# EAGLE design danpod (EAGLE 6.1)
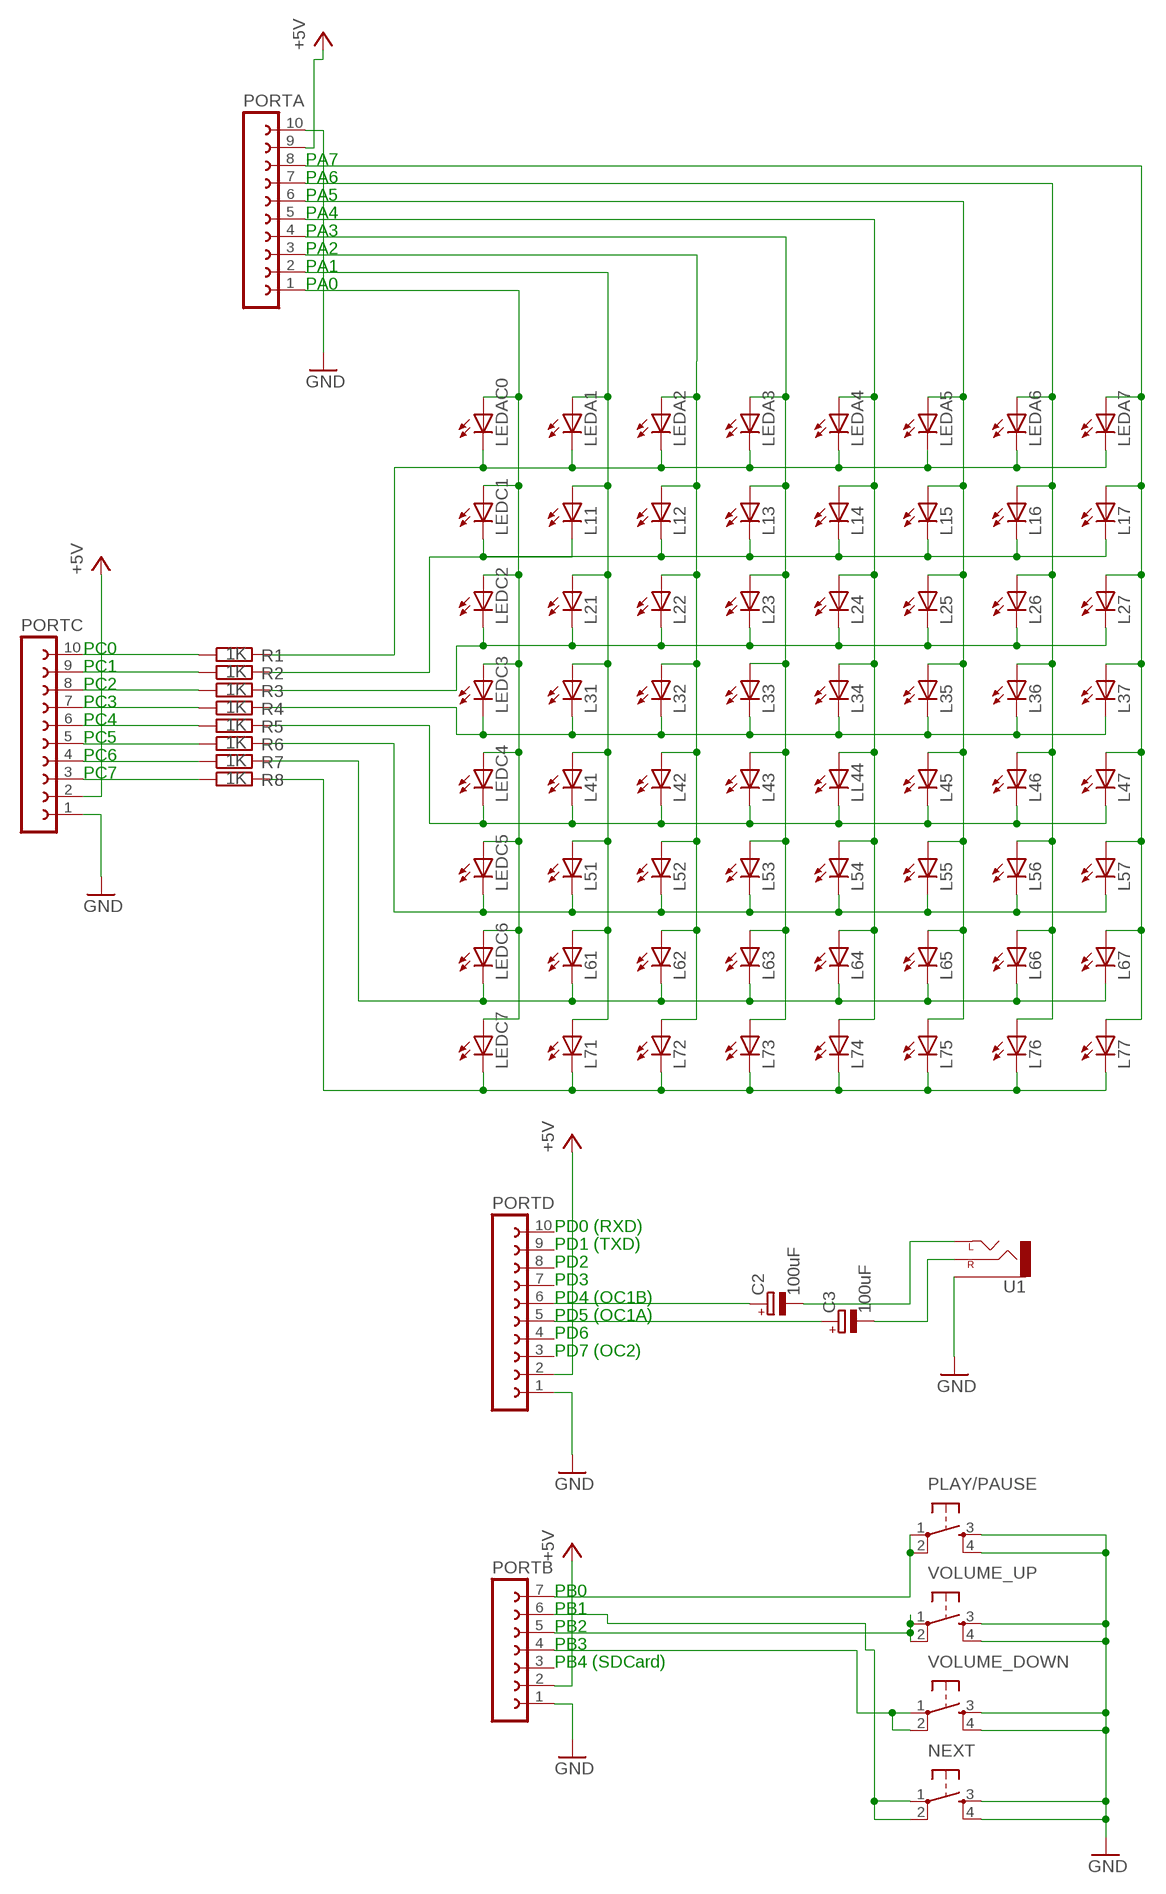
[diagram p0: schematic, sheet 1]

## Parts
C2  100uF  CPOL-EUE2,5-6E  [E2,5-6E]
C3  100uF  CPOL-EUE2,5-6E  [E2,5-6E]
L11  LED3MM  [LED3MM]
L12  LED3MM  [LED3MM]
L13  LED3MM  [LED3MM]
L14  LED3MM  [LED3MM]
L15  LED3MM  [LED3MM]
L16  LED3MM  [LED3MM]
L17  LED3MM  [LED3MM]
L21  LED3MM  [LED3MM]
L22  LED3MM  [LED3MM]
L23  LED3MM  [LED3MM]
L24  LED3MM  [LED3MM]
L25  LED3MM  [LED3MM]
L26  LED3MM  [LED3MM]
L27  LED3MM  [LED3MM]
L31  LED3MM  [LED3MM]
L32  LED3MM  [LED3MM]
L33  LED3MM  [LED3MM]
L34  LED3MM  [LED3MM]
L35  LED3MM  [LED3MM]
L36  LED3MM  [LED3MM]
L37  LED3MM  [LED3MM]
L41  LED3MM  [LED3MM]
L42  LED3MM  [LED3MM]
L43  LED3MM  [LED3MM]
L45  LED3MM  [LED3MM]
L46  LED3MM  [LED3MM]
L47  LED3MM  [LED3MM]
L51  LED3MM  [LED3MM]
L52  LED3MM  [LED3MM]
L53  LED3MM  [LED3MM]
L54  LED3MM  [LED3MM]
L55  LED3MM  [LED3MM]
L56  LED3MM  [LED3MM]
L57  LED3MM  [LED3MM]
L61  LED3MM  [LED3MM]
L62  LED3MM  [LED3MM]
L63  LED3MM  [LED3MM]
L64  LED3MM  [LED3MM]
L65  LED3MM  [LED3MM]
L66  LED3MM  [LED3MM]
L67  LED3MM  [LED3MM]
L71  LED3MM  [LED3MM]
L72  LED3MM  [LED3MM]
L73  LED3MM  [LED3MM]
L74  LED3MM  [LED3MM]
L75  LED3MM  [LED3MM]
L76  LED3MM  [LED3MM]
L77  LED3MM  [LED3MM]
LEDA1  LED3MM  [LED3MM]
LEDA2  LED3MM  [LED3MM]
LEDA3  LED3MM  [LED3MM]
LEDA4  LED3MM  [LED3MM]
LEDA5  LED3MM  [LED3MM]
LEDA6  LED3MM  [LED3MM]
LEDA7  LED3MM  [LED3MM]
LEDAC0  LED3MM  [LED3MM]
LEDC1  LED3MM  [LED3MM]
LEDC2  LED3MM  [LED3MM]
LEDC3  LED3MM  [LED3MM]
LEDC4  LED3MM  [LED3MM]
LEDC5  LED3MM  [LED3MM]
LEDC6  LED3MM  [LED3MM]
LEDC7  LED3MM  [LED3MM]
LL44  LED3MM  [LED3MM]
NEXT  TAC_SWITCHPTH  [TACTILE-PTH]
PLAY/PAUSE  TAC_SWITCHPTH  [TACTILE-PTH]
PORTA  FE10-1  [FE10]
PORTB  FE07-1  [FE07]
PORTC  FE10-1  [FE10]
PORTD  FE10-1  [FE10]
R1  1K  R-EU_0204/7  [0204/7]
R2  1K  R-EU_0204/7  [0204/7]
R3  1K  R-EU_0204/7  [0204/7]
R4  1K  R-EU_0204/7  [0204/7]
R5  1K  R-EU_0204/7  [0204/7]
R6  1K  R-EU_0204/7  [0204/7]
R7  1K  R-EU_0204/7  [0204/7]
R8  1K  R-EU_0204/7  [0204/7]
U1  AUDIO-JACKPTH  [AUDIO-JACK]
VOLUME_DOWN  TAC_SWITCHPTH  [TACTILE-PTH]
VOLUME_UP  TAC_SWITCHPTH  [TACTILE-PTH]

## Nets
A3: L13.A L23.A L33.A L43.A L53.A L63.A L73.A LEDA3.A PORTA.4
GND: NEXT.3 NEXT.4 PLAY/PAUSE.3 PLAY/PAUSE.4 PORTA.10 PORTB.1 PORTC.1 PORTD.1 U1.SLEEVE VOLUME_DOWN.3 VOLUME_DOWN.4 VOLUME_UP.3 VOLUME_UP.4
N$1: C3.- U1.RING(RIGHT)
N$2: LEDAC0.A LEDC1.A LEDC2.A LEDC3.A LEDC4.A LEDC5.A LEDC6.A LEDC7.A PORTA.1
N$3: L11.A L21.A L31.A L41.A L51.A L61.A L71.A LEDA1.A PORTA.2
N$4: L12.A L22.A L32.A L42.A L52.A L62.A L72.A LEDA2.A PORTA.3
N$5: C2.+ PORTD.6
N$6: L14.A L24.A L34.A L54.A L64.A L74.A LEDA4.A LL44.A PORTA.5
N$7: L15.A L25.A L35.A L45.A L55.A L65.A L75.A LEDA5.A PORTA.6
N$8: L16.A L26.A L36.A L46.A L56.A L66.A L76.A LEDA6.A PORTA.7
N$9: L17.A L27.A L37.A L47.A L57.A L67.A L77.A LEDA7.A PORTA.8
N$10: C2.- U1.TIP(LEFT)
N$11: L61.K(C) L62.K(C) L63.K(C) L64.K(C) L65.K(C) L66.K(C) L67.K(C) LEDC6.K(C) R7.2
N$12: L51.K(C) L52.K(C) L53.K(C) L54.K(C) L55.K(C) L56.K(C) L57.K(C) LEDC5.K(C) R6.2
N$13: L41.K(C) L42.K(C) L43.K(C) L45.K(C) L46.K(C) L47.K(C) LEDC4.K(C) LL44.K(C) R5.2
N$14: L31.K(C) L32.K(C) L33.K(C) L34.K(C) L35.K(C) L36.K(C) L37.K(C) LEDC3.K(C) R4.2
N$15: C3.+ PORTD.5
N$17: LEDA1.K(C) LEDA2.K(C) LEDA3.K(C) LEDA4.K(C) LEDA5.K(C) LEDA6.K(C) LEDA7.K(C) LEDAC0.K(C) R1.2
N$18: PORTC.4 R7.1
N$21: PLAY/PAUSE.1 PLAY/PAUSE.2 PORTB.7
N$22: PORTB.4 VOLUME_DOWN.1 VOLUME_DOWN.2
N$23: PORTB.5 VOLUME_UP.1 VOLUME_UP.2
N$24: NEXT.1 NEXT.2 PORTB.6
N$25: PORTC.3 R8.1
N$27: L71.K(C) L72.K(C) L73.K(C) L74.K(C) L75.K(C) L76.K(C) L77.K(C) LEDC7.K(C) R8.2
N$28: L21.K(C) L22.K(C) L23.K(C) L24.K(C) L25.K(C) L26.K(C) L27.K(C) LEDC2.K(C) R3.2
N$29: L11.K(C) L12.K(C) L13.K(C) L14.K(C) L15.K(C) L16.K(C) L17.K(C) LEDC1.K(C) R2.2
N$30: PORTC.5 R6.1
N$31: PORTC.6 R5.1
N$32: PORTC.7 R4.1
N$33: PORTC.8 R3.1
N$34: PORTC.9 R2.1
N$35: PORTC.10 R1.1
VCC: PORTA.9 PORTB.2 PORTC.2 PORTD.2 ; supply symbol labelled +5V
Unconnected: PORTB.3 PORTD.3 PORTD.4 PORTD.7 PORTD.8 PORTD.9 PORTD.10

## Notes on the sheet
- PA7
- PA6
- PA5
- PA4
- PA3
- PA2
- PA1
- PA0
- PC0
- PC1
- PC2
- PC3
- PC4
- PC5
- PC6
- PC7
- PD0 (RXD)
- PD1 (TXD)
- PD2
- PD3
- PD4 (OC1B)
- PD5 (OC1A)
- PD6
- PD7 (OC2)
- PB0
- PB1
- PB2
- PB3
- PB4 (SDCard)

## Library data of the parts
C2 C3 = rcl:CPOL-EU: POLARIZED CAPACITOR, European symbol
L11-L17 L21-L27 L31-L37 L41-L43 L45-L47 L51-L57 L61-L67 L71-L77 LEDA1-LEDA7 LEDAC0 LEDC1-LEDC7 LL44 = led:LED: LED
NEXT PLAY/PAUSE VOLUME_DOWN VOLUME_UP = SparkFun:TAC_SWITCH: Momentary Switch Button commonly used for reset or general input. Spark Fun Electronics SKU : COM-00097
PORTA PORTC PORTD = con-lsta:FE10-1: FEMALE HEADER; OC_FARNELL: unknown; OC_NEWARK: unknown
PORTB = con-lsta:FE07-1: FEMALE HEADER; OC_FARNELL: unknown; OC_NEWARK: unknown
R1-R8 = resistor:R-EU_: RESISTOR, European symbol
U1 = SparkFun:AUDIO-JACK: 3.5mm Audio Jack Simple 3.5mm common PCB mount audio jack. SKU: PRT-08032

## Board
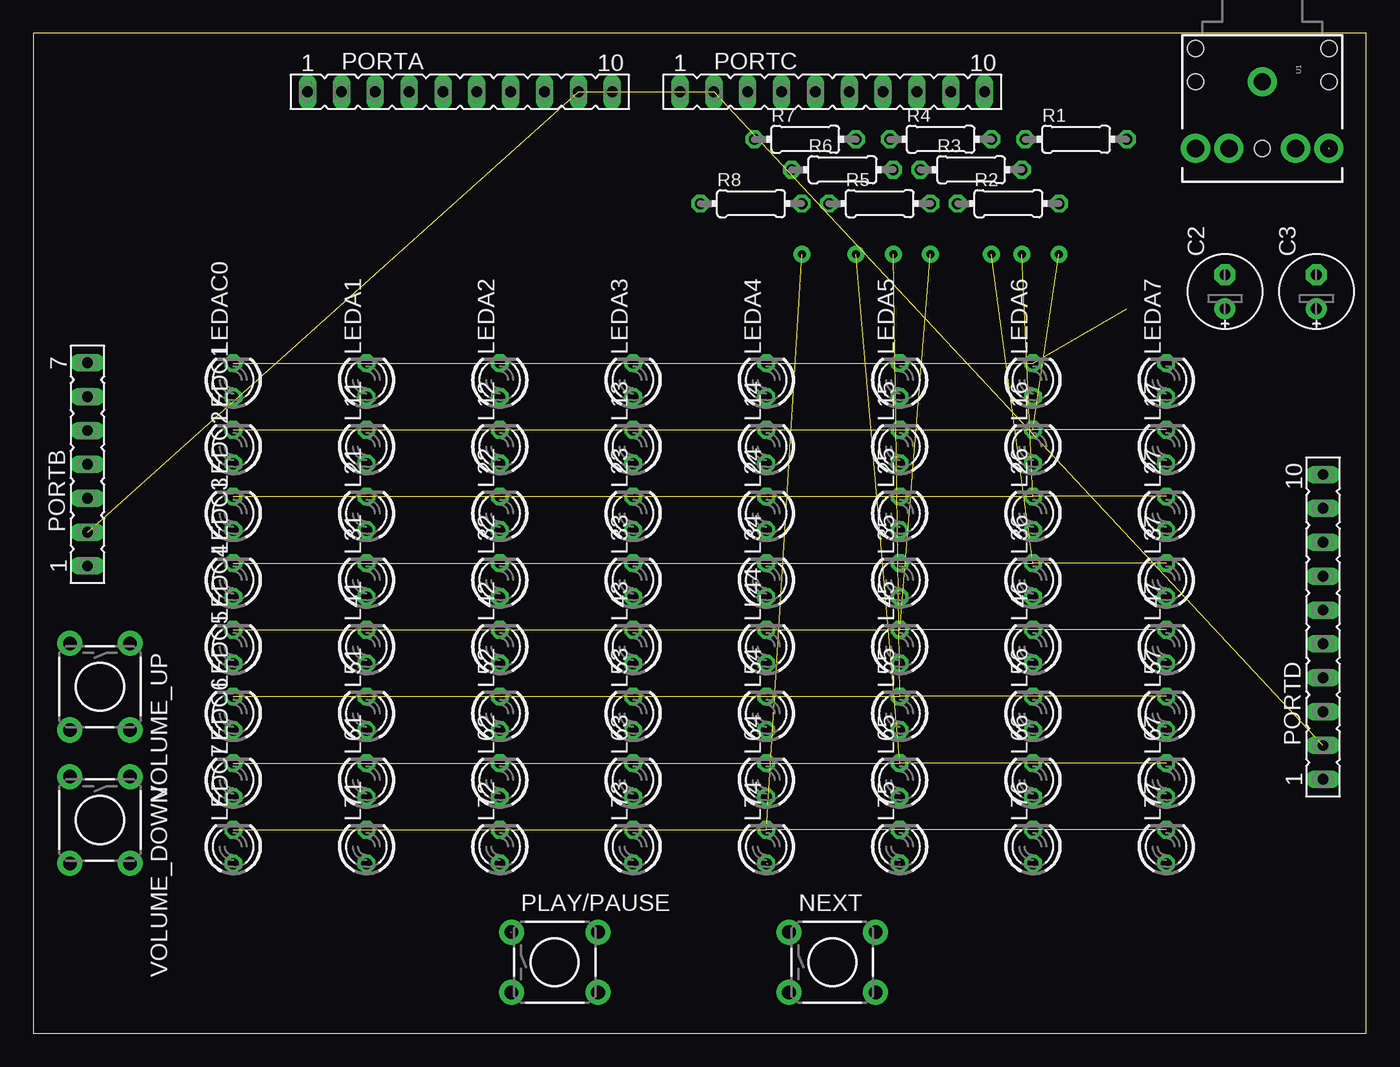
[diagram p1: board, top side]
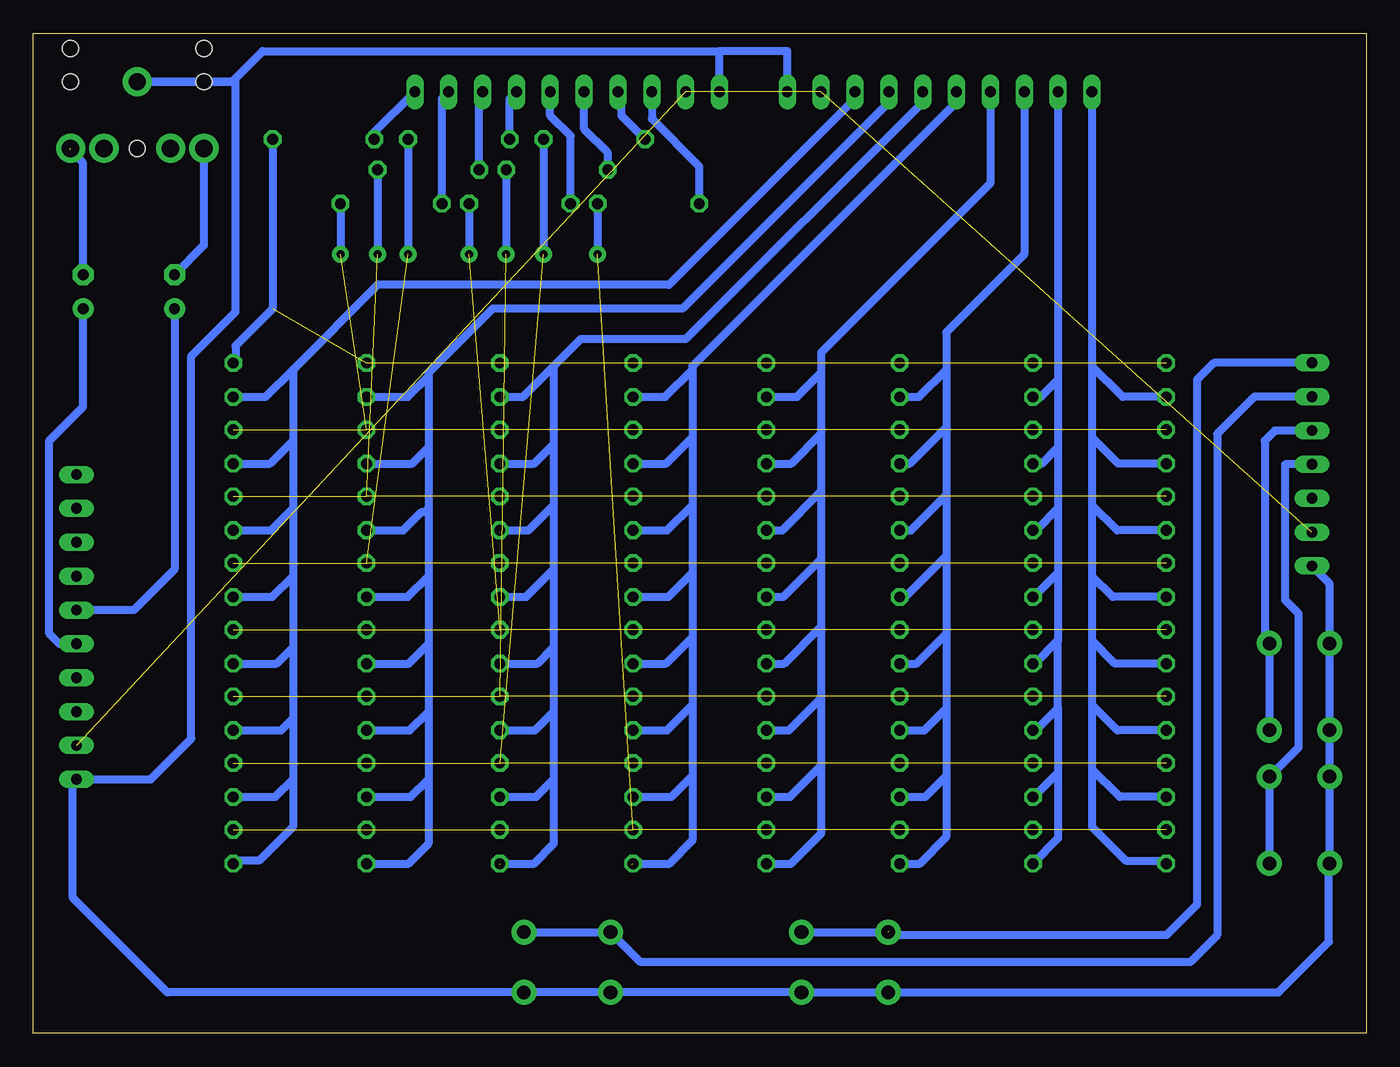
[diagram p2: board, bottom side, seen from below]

Size 100 x 75 mm. Coordinates in mm from the lower left corner, seen from the top.
Outline: 0,0 100,0 100,75 0,75 0,0
Copper layers (1*16): Top 0.035mm / dielectric 1.5mm / Bottom 0.035mm
Design rules: minimum track width 10mil, minimum drill 24mil, track to track 8mil, track to pad 8mil, pad to pad 8mil, via to via 8mil, smd to smd 8mil, copper to edge 40mil, drill to drill 8mil, minimum pad ring 10mil, minimum via ring 8mil, stop-mask expansion 4mil, vias tented up to drill 0mil, thermal gap 10mil

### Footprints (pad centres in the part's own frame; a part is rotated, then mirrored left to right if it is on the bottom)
E2,5-6E = drill 0.813 pad 1.575: + -1.27,0 | drill 0.813 pad 1.575 octagon: - 1.27,0
LED3MM = drill 0.813 octagon: A -1.27,0; K 1.27,0
TACTILE-PTH = drill 1.016 pad 1.88: 1 -3.251,2.261; 2 3.251,2.261; 3 -3.251,-2.261; 4 3.251,-2.261
FE10 = drill 0.813 long: 1 -11.43,0; 2 -8.89,0; 3 -6.35,0; 4 -3.81,0; 5 -1.27,0; 6 1.27,0; 7 3.81,0; 8 6.35,0; 9 8.89,0; 10 11.43,0
FE07 = drill 0.813 long: 1 -7.62,0; 2 -5.08,0; 3 -2.54,0; 4 0,0; 5 2.54,0; 6 5.08,0; 7 7.62,0
0204/7 = drill 0.813 octagon: 1 -3.81,0; 2 3.81,0
AUDIO-JACK = drill 1.3 pad 2.184: RING 5,5; RSH 5,2.5; SLEEVE 0,0; TIP 5,-5; TSH 5,-2.5 | hole 1.2: 0,5; -2.5,5; -2.5,-5; 0,-5; 5,0

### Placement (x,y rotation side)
C2  89.41,55.63 90 top
C3  96.27,55.63 90 top
L11  25,44 90 top
L12  35,44 90 top
L13  45,44 90 top
L14  55,44 90 top
L15  65,44 90 top
L16  75,44 90 top
L17  85,44 90 top
L21  25,39 90 top
L22  35,39 90 top
L23  45,39 90 top
L24  55,39 90 top
L25  65,39 90 top
L26  75,39 90 top
L27  85,39 90 top
L31  25,34 90 top
L32  35,34 90 top
L33  45,34 90 top
L34  55,34 90 top
L35  65,34 90 top
L36  75,34 90 top
L37  85,34 90 top
L41  25,29 90 top
L42  35,29 90 top
L43  45,29 90 top
L45  65,29 90 top
L46  75,29 90 top
L47  85,29 90 top
L51  25,24 90 top
L52  35,24 90 top
L53  45,24 90 top
L54  55,24 90 top
L55  65,24 90 top
L56  75,24 90 top
L57  85,24 90 top
L61  25,19 90 top
L62  35,19 90 top
L63  45,19 90 top
L64  55,19 90 top
L65  65,19 90 top
L66  75,19 90 top
L67  85,19 90 top
L71  25,14 90 top
L72  35,14 90 top
L73  45,14 90 top
L74  55,14 90 top
L75  65,14 90 top
L76  75,14 90 top
L77  85,14 90 top
LEDA1  25,49 90 top
LEDA2  35,49 90 top
LEDA3  45,49 90 top
LEDA4  55,49 90 top
LEDA5  65,49 90 top
LEDA6  75,49 90 top
LEDA7  85,49 90 top
LEDAC0  15,49 90 top
LEDC1  15,44 90 top
LEDC2  15,39 90 top
LEDC3  15,34 90 top
LEDC4  15,29 90 top
LEDC5  15,24 90 top
LEDC6  15,19 90 top
LEDC7  15,14 90 top
LL44  55,29 90 top
NEXT  59.94,5.33 0 top
PLAY/PAUSE  39.12,5.33 0 top
PORTA  32,70.61 0 top
PORTB  4.06,42.67 90 top
PORTC  59.94,70.61 0 top
PORTD  96.76,30.48 90 top
R1  78.23,67.06 0 top
R2  73.15,62.23 0 top
R3  70.36,64.77 0 top
R4  68.07,67.06 0 top
R5  63.5,62.23 0 top
R6  60.71,64.77 0 top
R7  57.91,67.06 0 top
R8  53.85,62.23 0 top
U1  92.2,71.37 270 top
VOLUME_DOWN  5,16 270 top
VOLUME_UP  5,26 270 top

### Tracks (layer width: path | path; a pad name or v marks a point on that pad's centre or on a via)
A3
  Bottom 0.61: PORTA.4 28.19,63.75 40.89,51.05 40.89,49.53 | 40.89,49.53 40.89,44.96 | 40.89,44.96 40.89,40.64 | 40.89,40.64 40.89,35.56 | 40.89,35.56 40.89,30.48 | 40.89,30.48 40.89,25.15 | 40.89,25.15 40.89,20.07 | 40.89,20.07 40.89,14.99 43.18,12.7 44.97,12.7 L73.A | L63.A 43.23,17.73 40.89,20.07 | L53.A 43.31,22.73 40.89,25.15 | L43.A 43.64,27.73 40.89,30.48 | L33.A 43.72,32.73 40.89,35.56 | L23.A 43.8,37.73 40.89,40.64 | L13.A 43.12,42.73 40.89,44.96 | LEDA3.A 42.69,47.73 40.89,49.53
GND
  Bottom 0.61: 48.51,73.66 82.8,73.66 85.09,71.37 U1.SLEEVE 84.84,71.37 84.84,54.1 88.14,50.8 88.14,22.1 91.19,19.05 PORTD.1 97.03,18.78 97.03,10.16 89.94,3.07 NEXT.4 NEXT.3 56.64,3.02 56.64,2.54 56.11,3.07 PLAY/PAUSE.4 PLAY/PAUSE.3 6.58,3.07 2.79,6.86 2.79,12.69 VOLUME_DOWN.4 VOLUME_DOWN.3 VOLUME_UP.4 VOLUME_UP.3 2.74,33.73 PORTB.1 | PORTC.1 48.51,73.66 | PORTA.10 43.43,73.66 48.51,73.66
N$1  (1 unrouted)
  Bottom 0.61: C3.- 96.27,65.28 97.28,66.29
N$2
  Bottom 0.61: PORTA.1 20.57,50.04 | 20.57,50.04 20.57,44.7 | 20.57,44.7 20.57,39.62 | 20.57,39.62 20.57,34.29 | 20.57,34.29 20.57,29.46 | 20.57,29.46 20.57,24.64 | 20.57,24.64 20.57,19.81 | 20.57,19.81 20.57,15.49 18.03,12.95 15.22,12.95 LEDC7.A | LEDC6.A 18.49,17.73 20.57,19.81 | LEDC5.A 18.67,22.73 20.57,24.64 | LEDC4.A 18.84,27.73 20.57,29.46 | LEDC3.A 19.01,32.73 20.57,34.29 | LEDC2.A 18.68,37.73 20.57,39.62 | LEDC1.A 18.6,42.73 20.57,44.7 | LEDAC0.A 18.27,47.73 20.57,50.04
N$3
  Bottom 0.61: PORTA.2 23.11,49.02 | 23.11,49.02 23.11,43.94 | 23.11,43.94 23.11,39.37 | 23.11,39.37 23.11,34.54 | 23.11,34.54 23.11,29.72 23.11,29.46 | 23.11,24.38 23.11,19.56 | 23.11,19.56 23.11,14.62 L71.A | L61.A 24.94,17.73 23.11,19.56 | L51.A 24.77,22.73 23.11,24.38 | L41.A 24.85,27.73 23.11,29.46 | L31.A 24.93,32.73 23.11,34.54 | L21.A 24.75,37.73 23.11,39.37 | L11.A 24.33,42.73 23.11,43.94 | LEDA1.A 24.41,47.73 23.11,49.02 | 23.11,24.38 23.11,29.46
N$4
  Bottom 0.61: PORTA.3 25.65,58.42 31.5,52.58 31.5,49.78 | 31.5,49.78 31.5,45.47 | 31.5,45.47 31.5,40.39 | 31.5,40.39 31.5,35.81 | 31.5,35.81 31.5,29.97 | 31.5,29.97 31.5,24.38 | 31.5,24.38 31.5,19.3 | 31.5,19.3 31.5,14.73 33.53,12.7 34.97,12.7 L72.A | L62.A 33.07,17.73 31.5,19.3 | L52.A 33.15,22.73 31.5,24.38 | L42.A 33.74,27.73 31.5,29.97 | L32.A 34.58,32.73 31.5,35.81 | L22.A 34.15,37.73 31.5,40.39 | L12.A 34.23,42.73 31.5,45.47 | LEDA2.A 33.55,47.73 31.5,49.78
N$5
  Bottom 0.61: PORTD.6 92.46,31.75 89.41,34.8 C2.+
N$6  (1 unrouted)
  Bottom 0.61: PORTA.5 30.73,69.85 50.55,50.04 50.55,49.78 | 50.55,49.78 50.55,44.7 | 50.55,44.7 50.55,39.62 | 50.55,39.62 50.55,34.54 | 50.55,34.54 50.55,29.72 | 50.55,29.72 50.55,24.64 | 50.55,24.64 50.55,19.3 | 50.55,19.3 50.55,14.48 52.32,12.7 55.12,12.7 54.86,12.95 | L64.A 52.12,17.73 50.55,19.3 | L54.A 52.45,22.73 50.55,24.64 | LL44.A 52.53,27.73 50.55,29.72 | L34.A 52.36,32.73 50.55,34.54 | L24.A 52.44,37.73 50.55,39.62 | L14.A 52.52,42.73 50.55,44.7 | LEDA4.A 52.6,47.73 50.55,49.78
N$7  (1 unrouted)
  Bottom 0.61: PORTA.6 33.27,69.85 51.05,52.07 58.93,52.07 60.96,50.04 | 60.96,50.04 60.96,44.2 | 60.96,44.2 60.96,39.62 | 60.96,39.62 60.96,34.8 | 60.96,34.8 60.96,28.96 | 60.96,28.96 60.96,24.13 | 60.96,24.13 60.96,19.05 | 60.96,19.05 60.96,14.22 62.48,12.7 65.02,12.7 | L65.A 62.28,17.73 60.96,19.05 | L55.A 62.36,22.73 60.96,24.13 | L45.A 62.19,27.73 60.96,28.96 | L35.A 63.03,32.73 60.96,34.8 | L25.A 62.85,37.73 60.96,39.62 | L15.A 62.43,42.73 60.96,44.2 | LEDA5.A 63.27,47.73 60.96,50.04
N$8
  Bottom 0.61: PORTA.7 35.81,69.85 51.31,54.36 65.53,54.36 70.36,49.53 70.36,49.28 | 70.36,49.28 70.36,43.94 | 70.36,43.94 70.36,39.37 | 70.36,39.37 70.36,34.29 | 70.36,34.29 70.36,29.21 | 70.36,29.21 70.36,24.13 | 70.36,24.13 70.36,19.05 | 70.36,19.05 70.36,14.22 71.88,12.7 74.97,12.7 L76.A | L66.A 71.68,17.73 70.36,19.05 | L56.A 71.76,22.73 70.36,24.13 | L46.A 71.84,27.73 70.36,29.21 | L36.A 71.92,32.73 70.36,34.29 | L26.A 72.25,37.73 70.87,39.12 70.61,39.12 70.36,39.37 | L16.A 71.57,42.73 70.36,43.94 | LEDA6.A 71.9,47.73 70.36,49.28
N$9
  Bottom 0.61: PORTA.8 38.35,70.1 52.32,56.13 74.17,56.13 80.52,49.78 | 80.52,49.78 80.52,44.45 | 80.52,44.45 80.52,39.37 | 80.52,39.37 80.52,34.29 | 80.52,34.29 80.52,28.96 | 80.52,28.96 80.52,23.62 | 80.52,23.62 80.52,19.05 | 80.52,19.05 80.52,15.49 83.06,12.95 84.78,12.95 L77.A | L67.A 81.84,17.73 80.52,19.05 | L57.A 81.41,22.73 80.52,23.62 | L47.A 81.74,27.73 80.52,28.96 | L37.A 82.08,32.73 80.52,34.29 | L27.A 82.16,37.73 80.52,39.37 | L17.A 82.24,42.73 80.52,44.45 | LEDA7.A 82.57,47.73 80.52,49.78
N$10
  Bottom 0.61: U1.TIP 87.2,59.1 C2.-
N$11  (via drill 0.6 pad 1.27)  (8 unrouted)
  Bottom 0.61: R7.2 v61.72,58.42
N$12  (via drill 0.6 pad 1.27)  (8 unrouted)
  Bottom 0.61: R6.2 v64.52,58.42
N$13  (via drill 0.6 pad 1.27)  (8 unrouted)
  Bottom 0.61: R5.2 v67.31,58.42
N$14  (via drill 0.6 pad 1.27)  (8 unrouted)
  Bottom 0.61: R4.2 v71.88,58.42
N$15
  Bottom 0.61: PORTD.5 98.04,29.21 98.81,29.97 98.81,44.45 96.27,46.99 C3.+
N$17  (7 unrouted)
  Bottom 0.61: R1.2 82.04,54.36 84.84,51.56 84.84,50.43 LEDA7.K
N$18
  Bottom 0.61: R7.1 55.88,68.83 55.88,70.36 PORTC.4
N$21  (1 unrouted)
  Bottom 0.61: PLAY/PAUSE.2 PLAY/PAUSE.1 | PORTB.7 11.43,50.29 12.7,49.02 12.7,9.65 14.99,7.37 35.56,7.37 35.81,7.62 | 35.81,7.62 36.07,7.87 36.07,7.62 35.81,7.62
N$22
  Bottom 0.61: PORTB.4 6.1,42.67 6.1,32.51 5.08,31.5 5.08,21.43 VOLUME_DOWN.1 VOLUME_DOWN.2
N$23
  Bottom 0.61: PORTB.5 6.86,45.21 7.62,44.45 7.62,29.61 VOLUME_UP.1 VOLUME_UP.2
N$24
  Bottom 0.61: NEXT.2 57.43,7.59 57.4,7.62 56.72,7.62 NEXT.1 54.43,5.33 13.21,5.33 11.18,7.37 11.18,44.96 8.38,47.75 PORTB.6
N$25
  Bottom 0.61: PORTC.3 53.59,68.58 50.04,65.02 R8.1
N$27  (via drill 0.6 pad 1.27)  (8 unrouted)
  Bottom 0.61: R8.2 v57.66,58.42
N$28  (via drill 0.6 pad 1.27)  (8 unrouted)
  Bottom 0.61: R3.2 v74.17,58.42
N$29  (via drill 0.6 pad 1.27)  (8 unrouted)
  Bottom 0.61: R2.2 v76.96,58.42
N$30
  Bottom 0.61: R6.1 56.9,66.04 58.67,67.82 PORTC.5
N$31
  Bottom 0.61: R5.1 59.69,67.31 61.21,68.83 PORTC.6
N$32
  Bottom 0.61: R4.1 64.26,70.1 PORTC.7
N$33
  Bottom 0.61: R3.1 66.55,70.36 PORTC.8
N$34
  Bottom 0.61: R2.1 69.34,70.1 PORTC.9
N$35
  Bottom 0.61: R1.1 74.42,67.56 PORTC.10
VCC  (3 unrouted)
